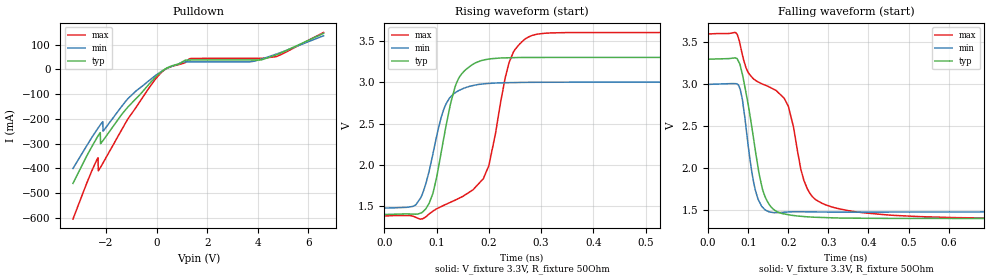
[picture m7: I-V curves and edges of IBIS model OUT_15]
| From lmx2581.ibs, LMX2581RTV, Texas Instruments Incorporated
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[Model]   OUT_15
Model_type   Open_drain
Polarity   Non-Inverting
Vmeas = 3.3
Vref = 3.3
Cref = 1pF
Rref = 50
|   typ   min   max
|   (nom PVT)   (slow PVT)   (fast PVT)
C_comp   0.269p   0.254p   0.289p
|C_comp (Hi state)   0.335p   0.327p   0.337p
|C_comp (Low state)   0.269p   0.254p   0.289p
[Voltage Range]   3.3   3   3.6
[Temperature Range]   27   125   -40
[Pullup Reference]   3.3   3   3.6
[Pulldown Reference]   0   0   0
[Power Clamp Reference]   3.3   3   3.6
[GND Clamp Reference]   0   0   0
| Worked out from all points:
|   slope of the pulldown table from 0 to 0.495 V, typ, clamps not added: 13.3 ohm
|   falling waveform, V_fixture 3.3V, R_fixture 50Ohm: 20-80 % time 40.4ps typ, 26.7ps min, 142ps max; typ from 3.3 V to 1.4 V
|   rising waveform, V_fixture 3.3V, R_fixture 50Ohm: 20-80 % time 36.7ps typ, 35.3ps min, 47.1ps max; typ from 1.4 V to 3.3 V
[Pulldown]
|   Voltage   I(typ)   I(min)   I(max)
-3.3V     -460.8mA   -400.7mA   -605.1mA
-2.33V    -272.2mA   -240.3mA   -360mA
-2.31V    -268.8mA   -237.3mA   -357.4mA
-2.3V     -267.2mA   -235.9mA   -409.9mA
-2.221V   -255.7mA   -224.4mA   -397.3mA
-2.211V   -300.1mA   -223mA     -395.6mA
-2.122V   -288.7mA   -211.6mA   -379.8mA
-2.112V   -287.4mA   -250mA     -378mA
293.7mV   -1.759mA   -2.305mA   -3.803mA
1.323V    37.91mA    30.35mA    43.51mA
4.739V    58.84mA    62.05mA    51.59mA
6.6V      145.8mA    136mA      149.3mA
[Ramp]
R_load = 50
|   typ   min   max
dV/dt_r   1.13842/3.67315e-11   0.911334/3.53335e-11   1.32909/4.70674e-11
dV/dt_f   1.13856/4.03907e-11   0.911261/2.66871e-11   1.32285/1.42376e-10
[Falling Waveform]
V_fixture = 3.3V
V_fixture_min = 3V
V_fixture_max = 3.6V
R_fixture = 50Ohm
C_fixture = 0F
|   Time   V(typ)   V(min)   V(max)
0s        3.3V       3V         3.6V
79.33ps   3.242V     2.952V     3.488V
100ps     2.76V      2.271V     3.141V
124.7ps   2.006V     1.63V      3.029V
143.6ps   1.646V     1.501V     2.988V
174.3ps   1.477V     1.472V     2.905V
200.1ps   1.447V     1.48V      2.74V
238.9ps   1.425V     1.482V     1.857V
286.2ps   1.414V     1.479V     1.579V
900ps     1.402V     1.481V     1.395V
[Rising Waveform]
V_fixture = 3.3V
V_fixture_min = 3V
V_fixture_max = 3.6V
R_fixture = 50Ohm
C_fixture = 0F
|   Time   V(typ)   V(min)   V(max)
0s        1.403V     1.481V     1.385V
60.32ps   1.406V     1.519V     1.368V
79.33ps   1.469V     1.771V     1.373V
92.98ps   1.655V     2.131V     1.443V
113.2ps   2.304V     2.661V     1.512V
137.3ps   2.976V     2.879V     1.581V
189.5ps   3.266V     2.979V     1.835V
238.9ps   3.295V     2.994V     3.239V
282.8ps   3.298V     2.998V     3.564V
900ps     3.3V       3V         3.6V
